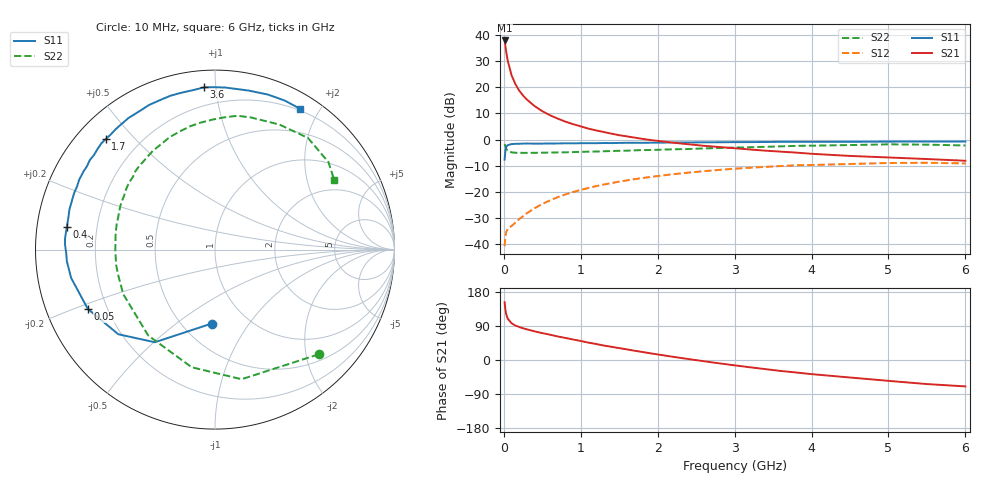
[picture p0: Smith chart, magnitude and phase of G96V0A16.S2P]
! SIEMENS Small Signal Semiconductors
! BFG235
! Si NPN RF Bipolar Junction Transistor in SOT223
! VCE = 6 V  IC = 160 mA
! Common Emitter S-Parameters:  July  1994
# GHz  S  MA  R  50
!  f  S11  S21  S12  S22
! GHz  MAG  ANG  MAG  ANG  MAG  ANG  MAG  ANG
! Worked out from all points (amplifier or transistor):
!   40 points, 10 MHz to 6 GHz, reference 50 ohm
!   highest |S21| = 38.0 dB at 10 MHz (marker M1)
!   |S21| within 3 dB of that: start of sweep to 24.31 MHz
!   unconditionally stable (mu >= 1): 452.4 MHz to 1.49 GHz
!   at 200 MHz: K = 0.81, MSG = 24.6 dB, |S12| = -30.5 dB
!   at 1.5 GHz: K = 1.00, MSG = 8.9 dB, |S12| = -16.2 dB
!   at 6 GHz: K = 0.89, MSG = 0.5 dB, |S12| = -9.2 dB
!   S11 on the Smith chart (normalised r, x): 10 MHz: 0.69, -0.68; 50 MHz: 0.13, -0.22; 400 MHz: 0.09, +0.08; 1.7 GHz: 0.08, +0.42; 3.6 GHz: 0.09, +0.93; 6 GHz: 0.18, +1.76
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0.01  0.4123 -92.5  79.68 152.4  0.009 64.0  0.821 -45.3
0.02  0.6154 -123.0  62.64 133.4  0.0139 49.3  0.7372 -78.4
0.03  0.7161 -138.8  49.12 121.6  0.0167 41.4  0.6683 -101.2
0.05  0.782 -155.0  32.68 109.0  0.0192 34.5  0.606 -127.9
0.1  0.8171 -168.9  17.25 97.0  0.022 37.0  0.5684 -154.1
0.15  0.8278 -175.4  11.59 90.9  0.0255 43.7  0.5577 -165.0
0.2  0.8294 -178.8  8.669 87.1  0.0298 48.0  0.5576 -171.1
0.25  0.8361 178.1  6.983 83.6  0.0338 51.8  0.5548 -175.3
0.3  0.8379 175.8  5.833 80.9  0.0386 54.8  0.5553 -178.9
0.4  0.8352 171.3  4.388 75.6  0.0481 57.3  0.5559 176.1
0.5  0.836 167.7  3.503 70.9  0.0581 58.5  0.5595 171.9
0.6  0.8412 164.7  2.927 66.8  0.0679 58.3  0.5632 167.9
0.7  0.8425 161.0  2.522 62.1  0.0785 57.9  0.5667 164.5
0.9  0.845 155.5  1.975 54.1  0.0983 55.1  0.5746 158.3
1.1  0.8521 149.2  1.619 45.8  0.1178 51.6  0.5854 152.1
1.7  0.8659 134.6  1.09 24.4  0.174 39.3  0.621 135.9
2.2  0.8774 123.3  0.871 8.4  0.2159 28.2  0.6499 122.3
3.2  0.8938 102.1  0.644 -19.2  0.2879 5.1  0.7119 96.5
3.6  0.9061 93.8  0.586 -28.9  0.3102 -4.8  0.7402 85.5
4.5  0.9056 78.1  0.485 -46.2  0.3395 -24.6  0.7838 62.7
5.5  0.9167 65.0  0.423 -63.5  0.3584 -46.6  0.798 37.6
6  0.9166 58.9  0.392 -69.7  0.3484 -54.8  0.7693 30.4
